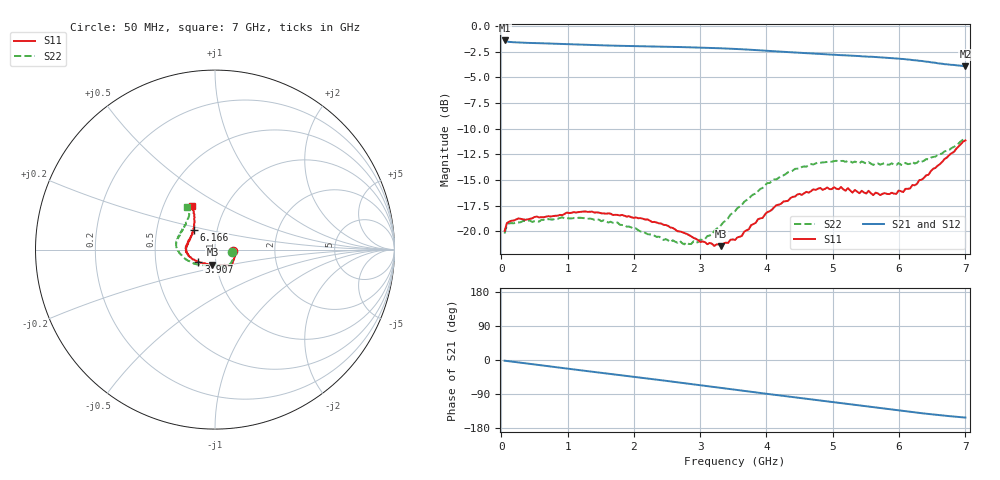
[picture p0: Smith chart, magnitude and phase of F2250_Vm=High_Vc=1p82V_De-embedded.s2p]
! Integrated Device Technology
! Corporate Headquarters
! 6024 Silver Creek Valley Road
! San Jose, CA 95138  USA
! Phone:  1-408-284-8200
! Toll Free:  1-800-223-1366
! Webpage:  http://www.idt.com/
! Timing and RF Division
! 515 Groton Road, Suite 102
! Westford, MA 01886-6024
! Device:  F2250
! Description: Voltage Variable RF Attenuator
! Frequency:  50.0 -  6000.00 MHz
! Package:  3x3 mm Thin QFN Plastic Package: 16 pin
! Ports:  2 RF, 3 DC
!  Pin  1  = GND
!  Pin  2  = NC
!  Pin  3  = RF1  = Port 1
!  Pin  4  = NC
!  Pin  5  = GND
!  Pin  6  = GND
!  Pin  7  = GND
!  Pin  8  = GND
!  Pin  9  = NC
!  Pin 10  = RF2  = Port 2
!  Pin 11  = NC
!  Pin 12  = GND
!  Pin 13  = GND
!  Pin 14  = VCNTRL
!  Pin 15  = VDD
!  Pin 16  = VMODE
! Vcntrl:  1.820 Volts
! Vmode:  +3.300 Volts
! Vdd:  +3.30  Volts
! Current:  1.325 mA
! Data:  The device was measured on a the F2250 evaluation board which has
!  individual transmission lines to the RF pins.  Data was collected
!  using a calibrated network analyzer.  The evaluation board was
!  de-embedded using a TRL calibration technique.
!  The reference plane is the edge of the package pin.
! Misc:  SN 10
!  Action Tracker AT0258
! Date Measured:  2014-11-26
! Date:  2015-10-15  MJV
! Note:
!  Integrated Device Technology supplies this data as a sample of measured
!  data at the package pin for this product.  Your particular data for this
!  product may vary.
!  Data was taken at 25 degrees C.
!  Integrated Device Technology reserves the right to change this data at anytime.
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# GHz S dB R 50
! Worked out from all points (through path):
!   201 points, 50 MHz to 7 GHz, reference 50 ohm
!   highest |S21| = -1.40 dB at 50 MHz (marker M1); lowest = -3.9 dB at 7 GHz (marker M2)
!   group delay of S21, straight-line fit = 61.1 ps
!   lowest |S11| = -21.4 dB at 3.317 GHz (marker M3), VSWR 1.19, Z = 47.9 - j8.06 ohm
!   |S11| at or under -10 dB: start of sweep to end of sweep
!   |S22| runs from -21.3 to -10.9 dB; largest |S21 - S12| = 0.0018
!   S11 on the Smith chart (normalised r, x): 50 MHz: 1.22, -0.02; 3.907 GHz: 0.82, -0.12; 6.166 GHz: 0.77, +0.17; 7 GHz: 0.69, +0.37
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0.05  -19.96 -5.5  -1.40 -1.8  -1.41 -1.8  -20.21 -6.7
0.08475  -19.20 -5.3  -1.51 -2.5  -1.51 -2.5  -19.40 -6.3
0.1195  -19.06 -6.0  -1.54 -3.3  -1.54 -3.3  -19.22 -6.4
0.71025  -18.52 -27.1  -1.70 -16.5  -1.70 -16.5  -18.81 -31.9
1.2315  -18.09 -41.7  -1.82 -27.9  -1.82 -27.9  -18.71 -51.3
1.75275  -18.40 -48.6  -1.92 -39.1  -1.92 -39.1  -19.14 -61.9
2.37825  -19.22 -51.8  -2.01 -52.6  -2.00 -52.6  -20.52 -72.2
2.552  -19.63 -55.2  -2.02 -56.4  -2.03 -56.5  -21.05 -78.7
2.86475  -20.49 -65.1  -2.07 -63.4  -2.07 -63.4  -21.23 -94.8
3.07325  -21.06 -78.1  -2.11 -68.1  -2.10 -68.1  -20.75 -109.5
3.3165  -21.45 -99.7  -2.17 -73.7  -2.16 -73.7  -19.38 -126.6
3.525  -20.84 -117.8  -2.23 -78.4  -2.23 -78.4  -18.04 -138.5
3.90725  -18.74 -143.4  -2.37 -87.0  -2.37 -87.0  -15.86 -156.9
4.1505  -17.45 -155.5  -2.47 -92.4  -2.47 -92.5  -14.93 -166.3
4.4285  -16.62 -165.4  -2.58 -98.6  -2.58 -98.6  -13.91 -175.0
4.7065  -15.91 -174.0  -2.68 -104.7  -2.68 -104.7  -13.48 178.4
5.1235  -15.68 175.3  -2.83 -113.9  -2.83 -113.9  -13.14 168.6
5.29725  -16.23 169.5  -2.89 -117.6  -2.88 -117.7  -13.31 165.3
5.85325  -16.37 150.1  -3.11 -129.8  -3.11 -129.9  -13.51 150.7
6.166  -15.82 137.1  -3.28 -136.6  -3.28 -136.7  -13.43 141.9
6.54825  -13.82 124.9  -3.58 -144.5  -3.58 -144.6  -12.72 129.6
7  -11.15 118.2  -3.91 -151.9  -3.91 -152.0  -10.94 122.7
